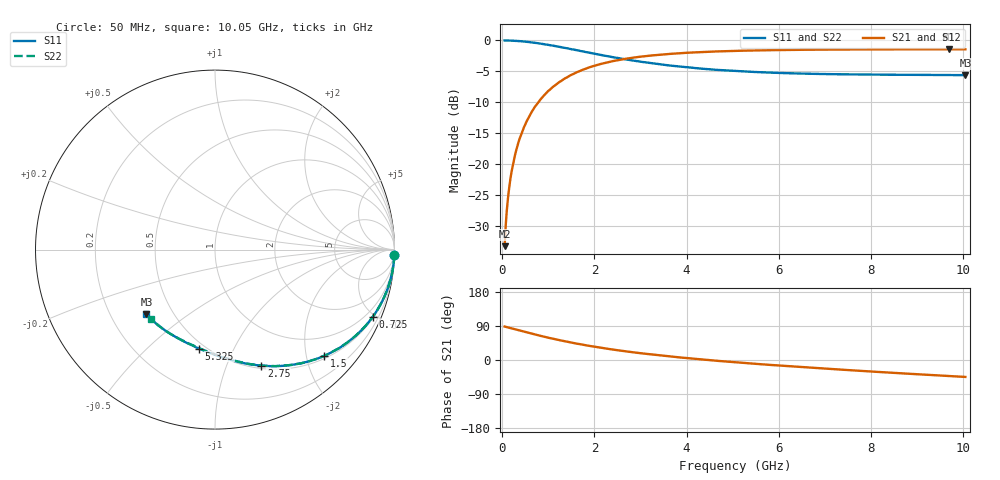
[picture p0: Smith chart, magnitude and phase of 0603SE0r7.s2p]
! AVX Thin Film Operation		Date: August 2001
! Description: Accu-P® Series, Thin Film, SMD, RF Capacitor
! Part Number: 06035J0R7ABT
! 50 MHz  -  10.05 GHz
! Serial Measurements
# mhz S db R 50
!	S11		S21		S12		S22
!	dB	Phase	dB	Phase	dB	Phase	dB	Phase
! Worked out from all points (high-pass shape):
!   401 points, 50 MHz to 10.05 GHz, reference 50 ohm
!   highest |S21| = -1.43 dB at 9.7 GHz (marker M1); lowest = -33.3 dB at 50 MHz (marker M2)
!   |S21| within 3 dB of the highest: 1.861 GHz to end of sweep
!   lowest |S11| = -5.6 dB at 10.05 GHz (marker M3), VSWR 3.20, Z = 17.8 - j17.6 ohm
!   |S11| at or under -10 dB: nowhere
!   |S22| runs from -5.6 to 0.0 dB; largest |S21 - S12| = 0
!   S11 on the Smith chart (normalised r, x): 50 MHz: 1, -69; 725 MHz: 0.56, -4.82; 1.5 GHz: 0.56, -2.36; 2.75 GHz: 0.53, -1.33; 5.325 GHz: 0.46, -0.74; 10.05 GHz: 0.36, -0.35
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50  -0.00 -1.6  -33.30 88.4  -33.30 88.4  -0.00 -1.6
75  -0.00 -2.5  -29.81 87.5  -29.81 87.5  -0.00 -2.5
125  -0.01 -4.1  -25.39 85.9  -25.39 85.9  -0.01 -4.1
175  -0.03 -5.8  -22.45 84.3  -22.45 84.3  -0.03 -5.8
225  -0.04 -7.4  -20.36 82.7  -20.36 82.7  -0.04 -7.4
300  -0.07 -9.8  -17.83 80.1  -17.83 80.1  -0.07 -9.8
375  -0.11 -12.3  -15.92 77.7  -15.92 77.7  -0.11 -12.3
475  -0.18 -15.4  -13.96 74.6  -13.96 74.6  -0.18 -15.4
725  -0.40 -23.2  -10.58 66.8  -10.58 66.8  -0.40 -23.2
1050  -0.78 -32.5  -7.85 57.5  -7.85 57.5  -0.78 -32.4
1500  -1.42 -44.1  -5.56 45.9  -5.56 45.9  -1.42 -44.1
1725  -1.75 -49.2  -4.80 40.8  -4.80 40.8  -1.75 -49.1
2250  -2.50 -59.8  -3.59 30.2  -3.59 30.2  -2.50 -59.7
2750  -3.15 -68.3  -2.89 21.7  -2.89 21.7  -3.15 -68.1
3400  -3.84 -77.7  -2.33 12.5  -2.33 12.5  -3.84 -77.2
4075  -4.40 -86.1  -1.97 4.2  -1.97 4.2  -4.39 -85.4
5050  -4.95 -96.5  -1.69 -6.0  -1.69 -6.0  -4.94 -95.3
5325  -5.05 -99.0  -1.64 -8.5  -1.64 -8.5  -5.04 -97.8
6725  -5.40 -111.9  -1.50 -20.7  -1.50 -20.7  -5.39 -109.0
8400  -5.55 -124.2  -1.45 -33.2  -1.45 -33.2  -5.52 -121.2
9700  -5.60 -134.1  -1.43 -42.3  -1.43 -42.3  -5.57 -130.1
10050  -5.61 -136.8  -1.43 -44.7  -1.43 -44.7  -5.58 -132.4
